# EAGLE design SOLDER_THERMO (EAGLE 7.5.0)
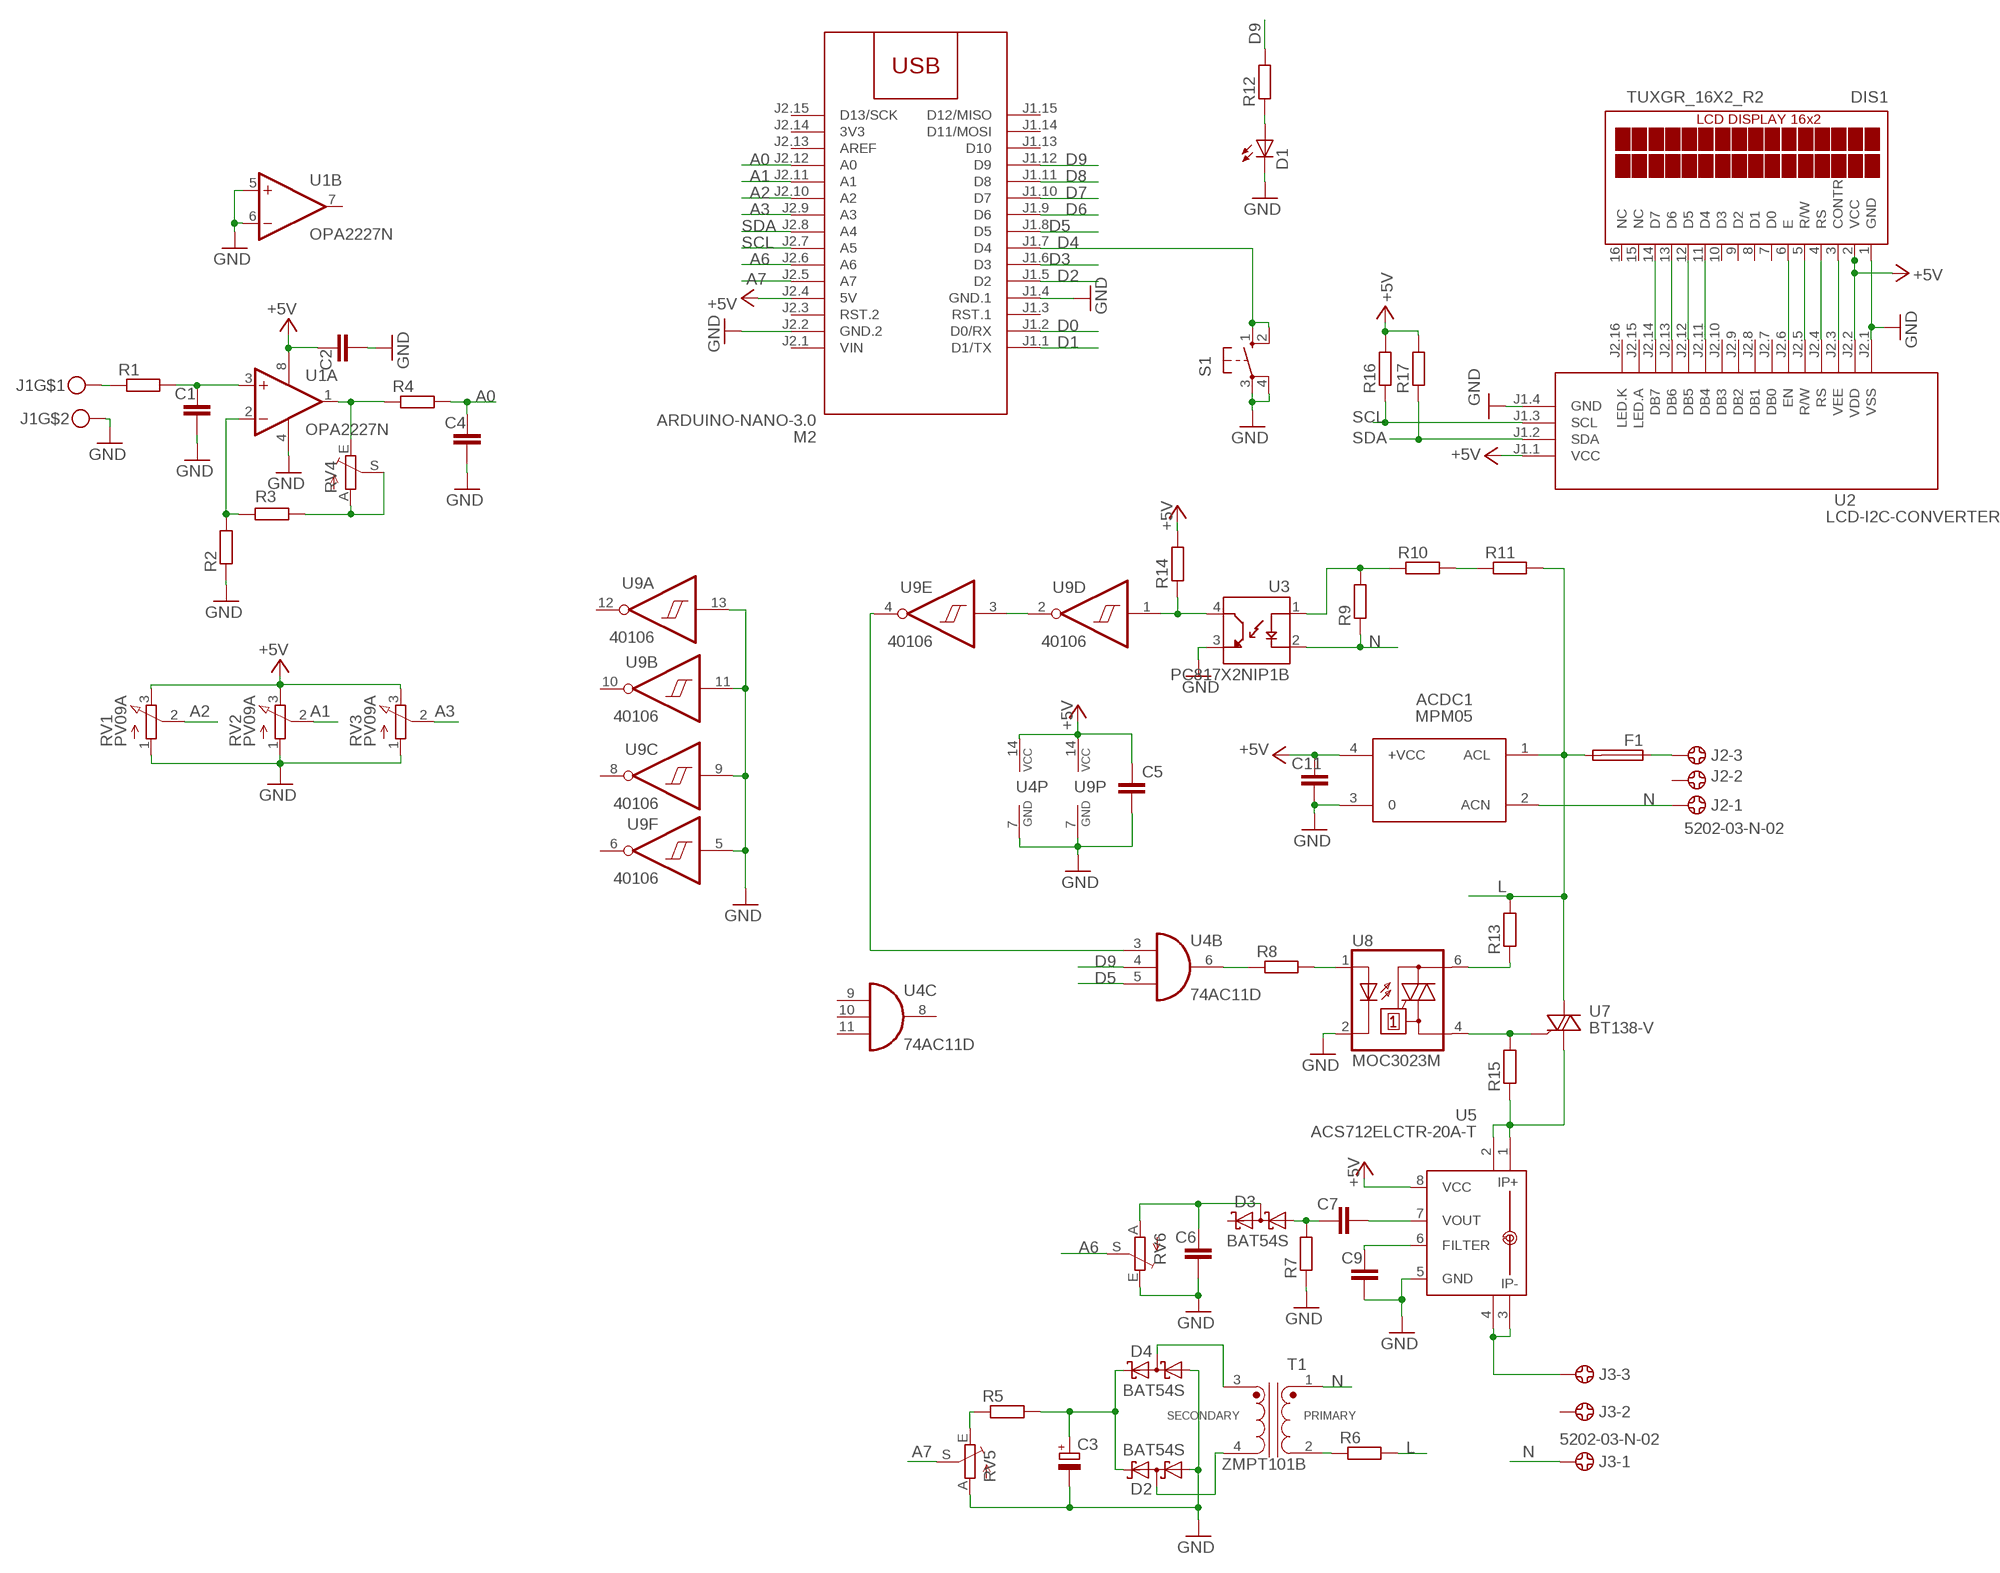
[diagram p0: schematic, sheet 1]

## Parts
ACDC1  MPM05  [MPM05]
C1  C-EUC1206  [C1206]
C2  C-EUC1206  [C1206]
C3  CPOL-EUSMCB  [SMC_B]
C4  C-EUC1206  [C1206]
C5  C-EUC1206  [C1206]
C6  C-EUC1206  [C1206]
C7  C-EUC1206  [C1206]
C9  C-EUC1206  [C1206]
C11  C-EUC1206  [C1206]
D1  LED5MM  [LED5MM]
D2  BAT54S  [SOT23]
D3  BAT54S  [SOT23]
D4  BAT54S  [SOT23]
DIS1  TUXGR_16X2_R2  [TUXGR_16X2_R2]
F1  FUSEBLANK_5X20MM  [FUSE_HOLDER_5X20MM]
J1  MKDSN1,5-2-5,08  [MKDSN1,5-2-5,08]
J2  5202-03-N-02  [5202-03-N-02]
J3  5202-03-N-02  [5202-03-N-02]
M2  ARDUINO-NANO-3.0  [ARDUINO-NANO-3.0]
R1  R-EU_R1206  [R1206]
R2  R-EU_R1206  [R1206]
R3  R-EU_R1206  [R1206]
R4  R-EU_R1206  [R1206]
R5  R-EU_R1206  [R1206]
R6  R-EU_0617/22  [0617/22]
R7  R-EU_R1206  [R1206]
R8  R-EU_R1206  [R1206]
R9  R-EU_R2512  [R2512]
R10  R-EU_R2512  [R2512]
R11  R-EU_R2512  [R2512]
R12  R-EU_R1206  [R1206]
R13  R-EU_R1206  [R1206]
R14  R-EU_R1206  [R1206]
R15  R-EU_R1206  [R1206]
R16  R-EU_R1206  [R1206]
R17  R-EU_R1206  [R1206]
RV1  PV09A  [PTV09]
RV2  PV09A  [PTV09]
RV3  PV09A  [PTV09]
RV4  TRIM_EU-B64W  [B64W]
RV5  TRIM_EU-B64W  [B64W]
RV6  TRIM_EU-B64W  [B64W]
S1  10-XX  [B3F-10XX]
T1  ZMPT101B  [XFMR_ZMPT101B]
U1  OPA2227N  [DIL08]
U2  LCD-I2C-CONVERTER  [LCD-I2C-CONVERTER]
U3  PC817X2NIP1B  [SOIC254P960X420-4N]
U4  74AC11D  [SO14]
U5  ACS712ELCTR-20A-T  [SO8]
U7  BT138-V  [TO220BV]
U8  MOC3023M  [DIL06]
U9  40106  74HC14D  [SO14]

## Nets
+5V: ACDC1.4(+VCC) C2.1 C5.1 C11.1 DIS1.2(VCC) M2.J2.4(5V) R14.2 R16.2 R17.2 RV1.3(E) RV2.3(E) RV3.3(E) U1.8(P:V+) U2.J1.1(VCC) U2.J2.2(VDD) U4.14(P:VCC) U5.8(VCC) U9.14(P:VCC)
A0: C4.1 M2.J2.12(A0) R4.2
A1: M2.J2.11(A1) RV2.2(S)
A2: M2.J2.10(A2) RV1.2(S)
A3: M2.J2.9(A3) RV3.2(S)
A6: M2.J2.6(A6) RV6.S
A7: M2.J2.5(A7) RV5.S
D0: M2.J1.2(D0/RX)
D1: M2.J1.1(D1/TX)
D2: M2.J1.5(D2)
D3: M2.J1.6(D3)
D4: M2.J1.7(D4) S1.1(S) S1.2(S1)
D5: M2.J1.8(D5) U4.5(B:I2)
D6: M2.J1.9(D6)
D7: M2.J1.10(D7)
D8: M2.J1.11(D8)
D9: M2.J1.12(D9) R12.2 U4.4(B:I1)
GND: ACDC1.3 C1.2 C2.2 C3.- C4.2 C5.2 C6.2 C9.2 C11.2 D1.K(C) D2.1(A1) D4.1(A1) DIS1.1(GND) J1.2 M2.J1.4(GND.1) M2.J2.2(GND.2) R2.1 R7.1 RV1.1(A) RV2.1(A) RV3.1(A) RV5.A RV6.E S1.3(P) S1.4(P1) U1.4(P:V-) U1.5(B:+IN) U1.6(B:-IN) U2.J1.4(GND) U2.J2.1(VSS) U3.3(ET) U4.7(P:GND) U5.5(GND) U8.2(C) U9.5(F:I) U9.7(P:GND) U9.9(C:I) U9.11(B:I) U9.13(A:I)
L: ACDC1.1(ACL) F1.2 R6.2 R11.2 R13.2 U7.T2(A2)
N: ACDC1.2(ACN) J2.1 J3.1 R9.1 T1.1 U3.2(C)
N$1: DIS1.14(D7) U2.J2.14(DB7)
N$2: DIS1.13(D6) U2.J2.13(DB6)
N$3: DIS1.12(D5) U2.J2.12(DB5)
N$4: DIS1.11(D4) U2.J2.11(DB4)
N$5: DIS1.6(E) U2.J2.6(EN)
N$6: DIS1.5(R/W) U2.J2.5(R/W)
N$7: DIS1.4(RS) U2.J2.4(RS)
N$8: R2.2 R3.2 U1.2(A:-IN)
N$9: C1.1 R1.2 U1.3(A:+IN)
N$10: DIS1.3(CONTR) U2.J2.3(VEE)
N$11: U9.2(D:O) U9.3(E:I)
N$12: R3.1 RV4.A RV4.S
N$13: R4.1 RV4.E U1.1(A:OUT)
N$14: J1.1 R1.1
N$15: R9.2 R10.1 U3.1(A)
N$16: R10.2 R11.1
N$17: R14.1 U3.4(CT) U9.1(D:I)
N$18: R8.2 U8.1(A)
N$19: F1.1 J2.3
N$20: R6.1 T1.2
N$21: R13.1 U8.6(A2)
N$23: R15.2 U7.G U8.4(A1)
N$24: R15.1 U5.1(IP+) U5.2(IP+1) U7.T1(A1)
N$25: R8.1 U4.6(B:O)
N$26: U4.3(B:I0) U9.4(E:O)
N$27: C9.1 U5.6(FILTER)
N$28: D4.3(C1A2) T1.3
N$29: D2.3(C1A2) T1.4
N$30: C3.+ D2.2(C2) D4.2(C2) R5.2
N$31: J3.3 U5.3(IP-) U5.4(IP-1)
N$32: C7.2 U5.7(VOUT)
N$33: C7.1 D3.1(A1) R7.2
N$34: C6.1 D3.3(C1A2) RV6.A
N$35: R5.1 RV5.E
N$37: D1.A R12.1
SCL: M2.J2.7(A5) R16.1 U2.J1.3(SCL)
SDA: M2.J2.8(A4) R17.1 U2.J1.2(SDA)
Unconnected: D3.2(C2) DIS1.7(D0) DIS1.8(D1) DIS1.9(D2) DIS1.10(D3) DIS1.15(NC) DIS1.16(NC) J2.2 J3.2 M2.J1.3(RST.1) M2.J1.13(D10) M2.J1.14(D11/MOSI) M2.J1.15(D12/MISO) M2.J2.3(RST.2) M2.J2.13(AREF) M2.J2.15(D13/SCK) U1.7(B:OUT) U2.J2.7(DB0) U2.J2.8(DB1) U2.J2.9(DB2) U2.J2.10(DB3) U2.J2.15(LED.A) U2.J2.16(LED.K) U4.1(A:I0) U4.2(A:I1) U4.8(C:O) U4.9(C:I0) U4.10(C:I1) U4.11(C:I2) U4.12(A:O) U4.13(A:I2) U9.6(F:O) U9.8(C:O) U9.10(B:O) U9.12(A:O)

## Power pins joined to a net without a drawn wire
3V3: M2.J2.14(3V3)
VIN: M2.J2.1(VIN)

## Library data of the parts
ACDC1 = acdc:MPM05: AC DC Converter 5W
C1 C2 C4-C7 C9 C11 = rcl:C-EU: CAPACITOR, European symbol
C3 = rcl:CPOL-EU: POLARIZED CAPACITOR, European symbol
D1 = led:LED: LED
D2-D4 = diode:BAT54S: Schottky Diodes Pin connection corrected 2011-05-04 Source: Fairchild .. BAT54.pdf
DIS1 = display-lcd:TUXGR_16X2_R2: Tuxgraphics LCD display 16x2 characters reflective, without background light Source: tuxgr_12x2_r2.pdf; OC_FARNELL: unknown; OC_NEWARK: unknown
F1 = fuse:FUSE: Fuse; OC_FARNELL: unknown; OC_NEWARK: unknown
J1 = con-phoenix-508:MKDSN1,5-2-5,08
J2 J3 = con-ebyelectro:5202-03-N-02: Barrier Blocks Sreies 5202 Source: http://www.ebyelectro.com/PDF/5202-XX-N-02.pdf; OC_FARNELL: unknown; OC_NEWARK: unknown
M2 = diy-modules:ARDUINO-NANO-3.0: Arduino Nano 3.0 and compatible devices More details available here: https://www.arduino.cc/en/Main/ArduinoBoardNano Click here to find device on ebay.com
R1-R17 = rcl:R-EU_: RESISTOR, European symbol
RV1-RV3 = pot:PV09A
RV4-RV6 = pot:TRIM_EU-: POTENTIOMETER
S1 = switch-omron:10-XX: OMRON SWITCH; MPN: B3F-1000; OC_FARNELL: 176432; OC_NEWARK: 36M3542
T1 = ZMPT101B:ZMPT101B: Check availability; AVAILABILITY: Not in stock; CHECK_PRICES: https://www.snapeda.com/parts/ZMPT101B/Qingxian+Zeming+Langxi+Electronic/view-part/?ref=eda; DESCRIPTION: Current-type Voltage Transformer; MF: Qingxian Zeming Langxi Electronic; MP: ZMPT101B; PACKAGE: None; PRICE: None; SNAPEDA_LINK: https://www.snapeda.com/parts/ZMPT101B/Qingxian+Zeming+Langxi+Electronic/view-part/?ref=snap
U1 = linear:OPA222*: High Precision, Low Noise OPERATIONAL AMPLIFIERS Source: http://focus.ti.com/lit/ds/symlink/opa227.pdf
U2 = diy-modules:LCD-I2C-CONVERTER: I2C Bus to 4-Bit Parallel LCD Interface with LED backlight driver
U3 = PC817X2NIP1B:PC817X2NIP1B: Check availability; AVAILABILITY: In Stock; CHECK_PRICES: https://www.snapeda.com/parts/PC817X2NIP1B/Sharp/view-part/?ref=eda; DESCRIPTION: Optocoupler DC-IN 1-CH Transistor DC-OUT 4-Pin DIP SMD T/R; MF: Sharp Microelectronics; MP: PC817X2NIP1B; PACKAGE: SMD-4 Sharp Microelectronics; PRICE: None; SNAPEDA_LINK: https://www.snapeda.com/parts/PC817X2NIP1B/Sharp/view-part/?ref=snap
U4 = 74xx-eu:74*11: Triple 3-input AND gate
U5 = allegro:ACS712ELCTR-20A-T: Fully Integrated, Hall Effect-Based Linear Current Sensor with High Voltage Isolation and a Low-Resistance Current Conductor.
U7 = triac:BT138: TRIAC Source: http://www.semiconductors.philips.com BT138_SERIES_2.pdf
U8 = optocoupler:MOC30*M: RANDOM-PHASE OPTOISOLATORS TRIAC DRIVER OUTPUT Source: http://www.fairchildsemi.com MOC3020-M.pdf; MF: FAIRCHILD SEMICONDUCTOR; MPN: MOC3023-M; OC_FARNELL: 1021367; OC_NEWARK: 72K8896
U9 = 74xx-eu:74*14: Hex schmitt trigger INVERTER

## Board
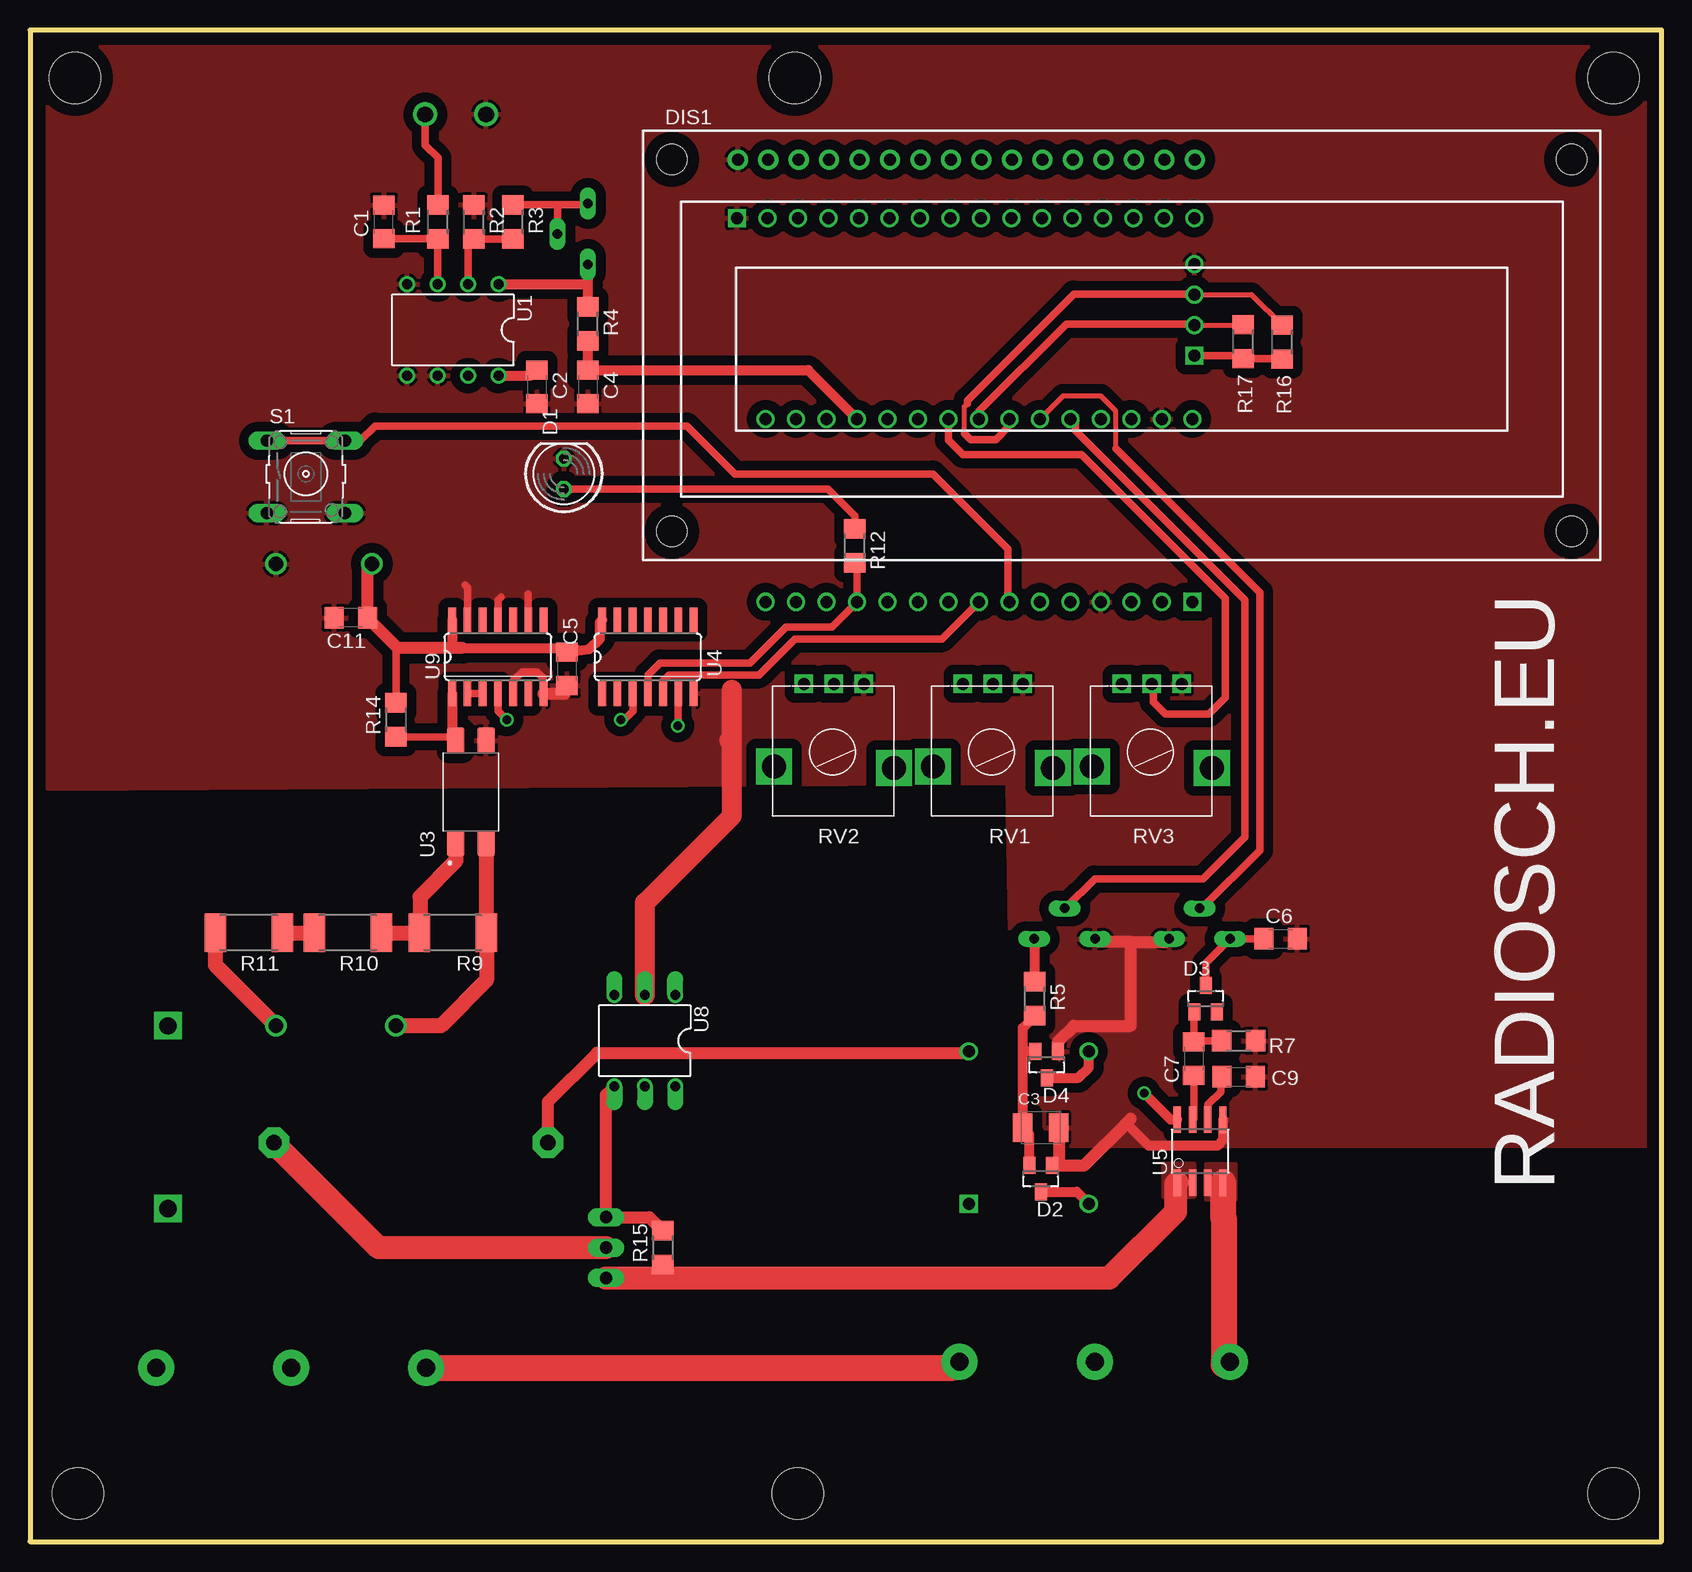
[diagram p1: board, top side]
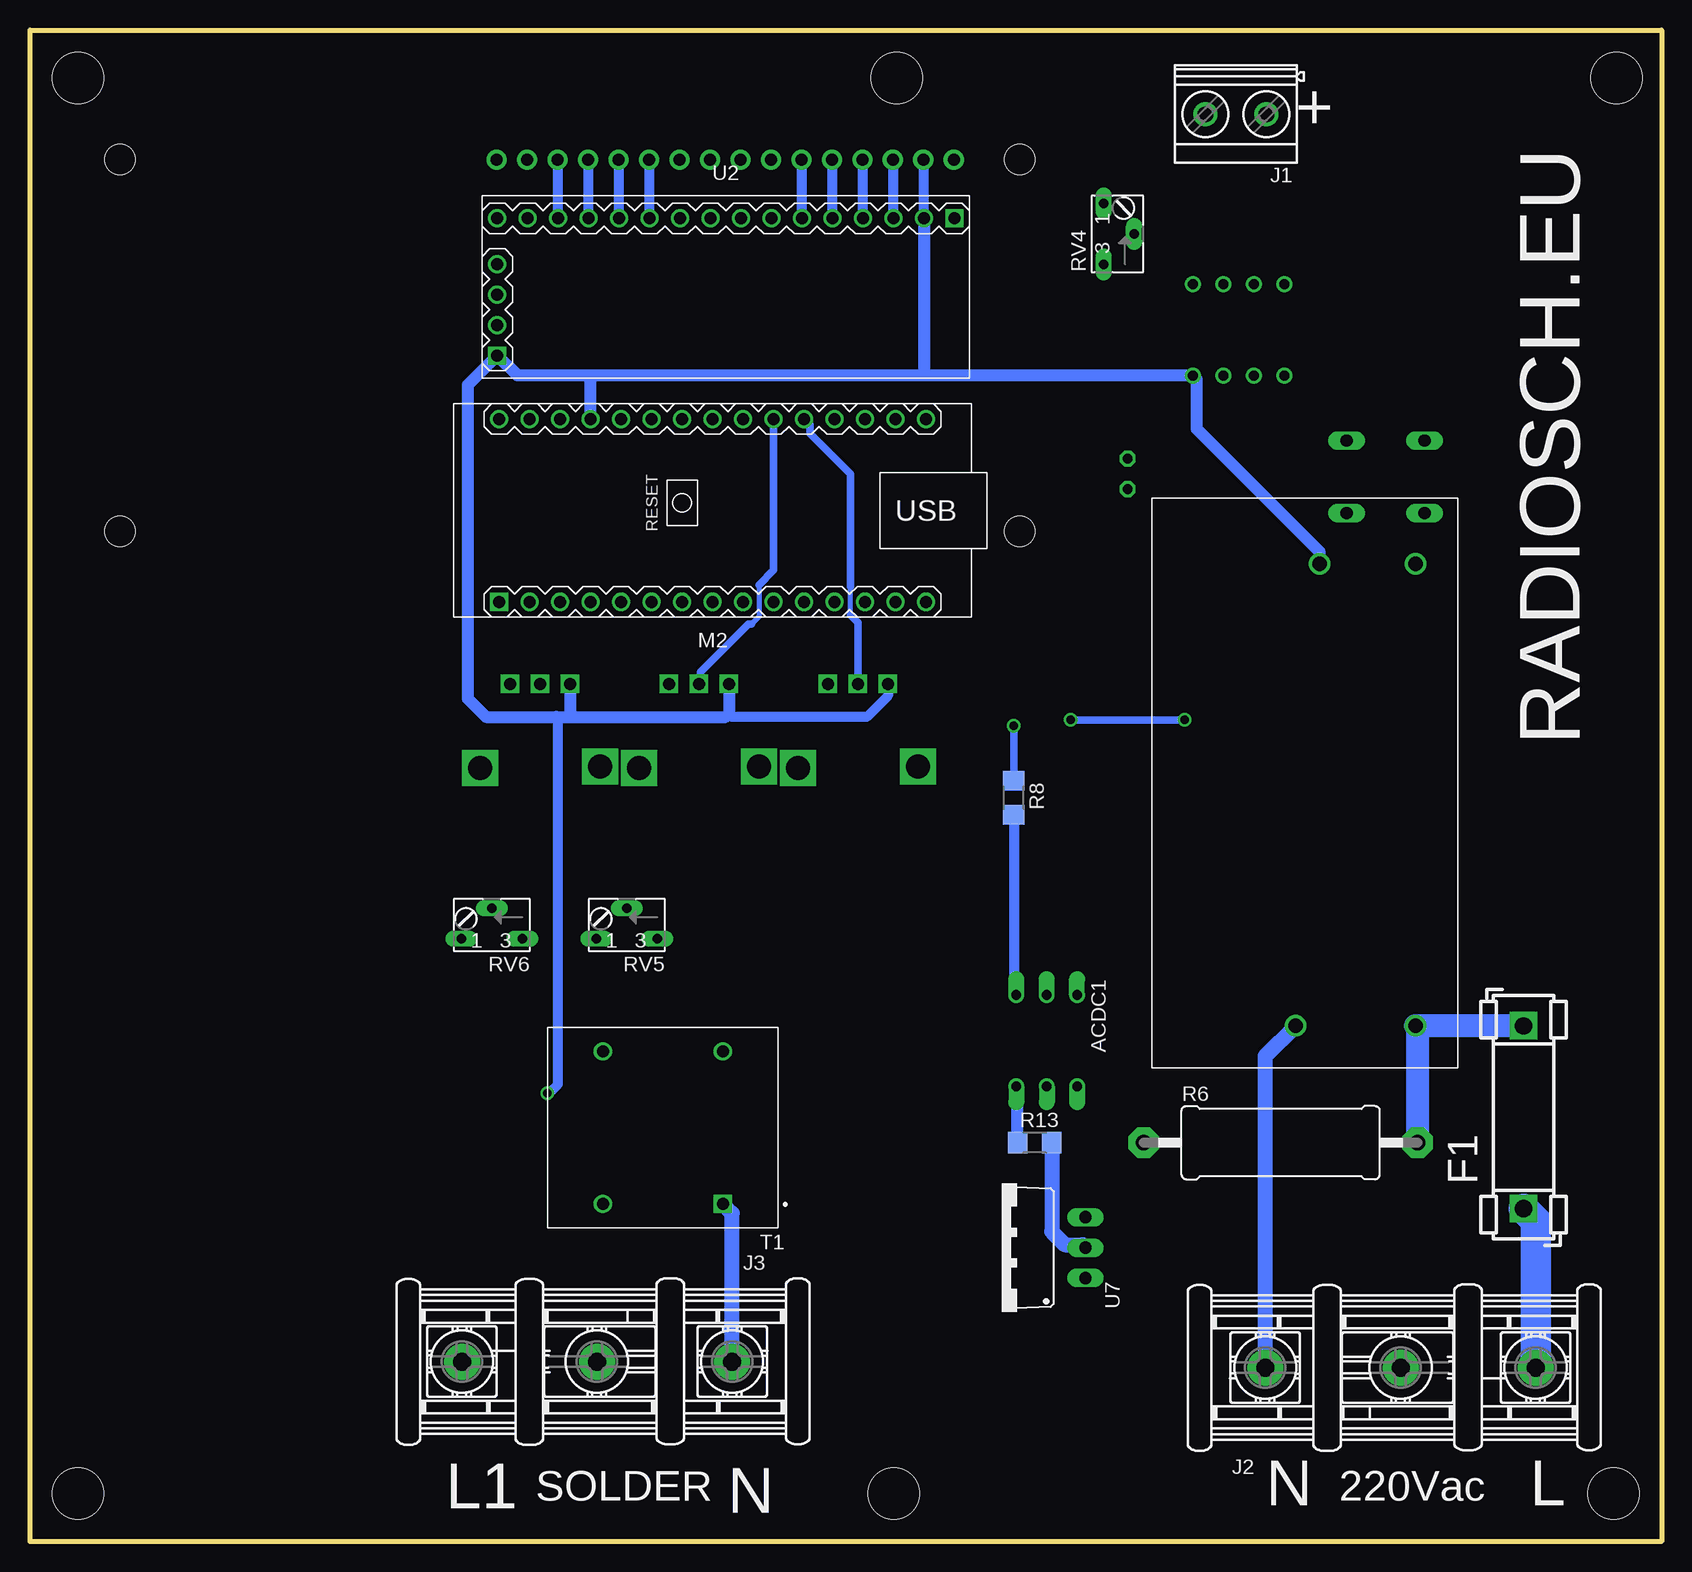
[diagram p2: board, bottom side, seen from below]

Size 136 x 126 mm. Coordinates in mm from the lower left corner, seen from the top.
Outline: 0,0 136,0 136,126 0,126 0,0
Copper layers (1*16): Top 0.035mm / dielectric 1.5mm / Bottom 0.035mm
Design rules "default *": minimum track width 10mil, minimum drill 24mil, track to track 4mil, track to pad 6mil, pad to pad 4mil, via to via 8mil, smd to smd 8mil, copper to edge 40mil, drill to drill 8mil, minimum pad ring 10mil, minimum via ring 8mil, stop-mask expansion 4mil, vias tented up to drill 0mil, thermal gap 10mil
Holes 4.3 mm at 3.75,122 4,4 132,4 132,122 64,4 63.75,122

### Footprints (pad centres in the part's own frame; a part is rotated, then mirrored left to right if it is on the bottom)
MPM05 = drill 1.2: 1 3.5,-22; 2 3.5,-12; 3 42,-22; 4 42,-14
C1206 = smd 1.6 x 1.8: 1 -1.4,0; 2 1.4,0
SMC_B = smd 1.6 x 2.4: + -1.5,0; - 1.5,0
LED5MM = drill 0.813 octagon: A -1.27,0; K 1.27,0
SOT23 = smd 1 x 1.4: 1 -0.95,-1.1; 2 0.95,-1.1; 3 0,1.1
TUXGR_16X2_R2 = drill 1 pad 1.676: 1 -32,15.5; 2 -29.46,15.5; 3 -26.92,15.5; 4 -24.38,15.5; 5 -21.84,15.5; 6 -19.3,15.5; 7 -16.76,15.5; 8 -14.22,15.5; 9 -11.68,15.5; 10 -9.14,15.5; 11 -6.6,15.5; 12 -4.06,15.5; 13 -1.52,15.5; 14 1.02,15.5; 15 3.56,15.5; 16 6.1,15.5 | hole 2.5: -37.5,-15.5; 37.5,-15.5; -37.5,15.5; 37.5,15.5
FUSE_HOLDER_5X20MM = drill 1.422 pad 2.286 square: 1 0,0; 2 15.24,0
MKDSN1,5-2-5,08 = drill 1.3 pad 2: 1 -2.561,0.025; 2 2.519,0.025
5202-03-N-02 = drill 1.5 pad 3: 1 -9.29,0; 2 2,0; 3 13.25,0
ARDUINO-NANO-3.0 = drill 1 square: J1.1 17.78,7.62 | drill 1: J1.2 15.24,7.62; J1.3 12.7,7.62; J1.4 10.16,7.62; J1.5 7.62,7.62; J1.6 5.08,7.62; J1.7 2.54,7.62; J1.8 0,7.62; J1.9 -2.54,7.62; J1.10 -5.08,7.62; J1.11 -7.62,7.62; J1.12 -10.16,7.62; J1.13 -12.7,7.62; J1.14 -15.24,7.62; J1.15 -17.78,7.62; J2.1 17.78,-7.62; J2.2 15.24,-7.62; J2.3 12.7,-7.62; J2.4 10.16,-7.62; J2.5 7.62,-7.62; J2.6 5.08,-7.62; J2.7 2.54,-7.62; J2.8 0,-7.62; J2.9 -2.54,-7.62; J2.10 -5.08,-7.62; J2.11 -7.62,-7.62; J2.12 -10.16,-7.62; J2.13 -12.7,-7.62; J2.14 -15.24,-7.62; J2.15 -17.78,-7.62
R1206 = smd 1.6 x 1.803: 1 -1.422,0; 2 1.422,0
0617/22 = drill 1.3 pad 2.54 octagon: 1 -11.43,0; 2 11.43,0
R2512 = smd 1.8 x 3.2: 1 -2.8,0; 2 2.8,0
PTV09 = drill 1 square: 1 -2.5,0; 2 0,0; 3 2.5,0 | drill 2 square: P$4 -5,7; P$5 5,6.9
B64W = drill 0.813 long: A 2.54,0; E -2.54,0; S 0,-2.54
B3F-10XX = drill 1.016 long: 1 -3.251,2.761; 2 3.251,2.761; 3 -3.251,-3.261; 4 3.251,-3.261
XFMR_ZMPT101B = drill 1 square: 1 -5,6.35 | drill 1: 2 -5,-6.35; 3 5,-6.35; 4 5,6.35
DIL08 = drill 0.813 pad 1.27: 1 -3.81,-3.81; 2 -1.27,-3.81; 3 1.27,-3.81; 4 3.81,-3.81; 5 3.81,3.81; 6 1.27,3.81; 7 -1.27,3.81; 8 -3.81,3.81
LCD-I2C-CONVERTER = drill 1 square: J1.1 -19.05,-5.08; J2.1 19.05,6.35 | drill 1: J1.2 -19.05,-2.54; J1.3 -19.05,0; J1.4 -19.05,2.54; J2.2 16.51,6.35; J2.3 13.97,6.35; J2.4 11.43,6.35; J2.5 8.89,6.35; J2.6 6.35,6.35; J2.7 3.81,6.35; J2.8 1.27,6.35; J2.9 -1.27,6.35; J2.10 -3.81,6.35; J2.11 -6.35,6.35; J2.12 -8.89,6.35; J2.13 -11.43,6.35; J2.14 -13.97,6.35; J2.15 -16.51,6.35; J2.16 -19.05,6.35
SOIC254P960X420-4N = smd 2.15 x 1.48: 1 -4.28,1.27; 2 -4.28,-1.27; 3 4.28,-1.27; 4 4.28,1.27
SO14 = smd 0.66 x 2.032: 1 -3.81,-3.073; 2 -2.54,-3.073; 3 -1.27,-3.073; 4 0,-3.073; 5 1.27,-3.073; 6 2.54,-3.073; 7 3.81,-3.073; 8 3.81,3.073; 9 2.54,3.073; 10 1.27,3.073; 11 0,3.073; 12 -1.27,3.073; 13 -2.54,3.073; 14 -3.81,3.073
SO8 = smd 0.61 x 2.21: 1 0.635,-0.076; 2 1.905,-0.076; 3 3.175,-0.076; 4 4.445,-0.076; 5 4.445,5.156; 6 3.175,5.156; 7 1.905,5.156; 8 0.635,5.156
TO220BV = drill 1.016 long: G 2.54,-6.985; T1 -2.54,-6.985; T2 0,-6.985
DIL06 = drill 0.813 offset: 1 -2.54,-3.81; 2 0,-3.81; 3 2.54,-3.81; 4 2.54,3.81; 5 0,3.81; 6 -2.54,3.81

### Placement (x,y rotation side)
ACDC1  42.5,39.5 90 bottom
C1  29.5,110 90 top
C2  42.25,96.25 270 top
C3  84.25,34.5 0 top
C4  46.5,96.25 270 top
C5  44.75,72.75 270 top
C6  104.25,50.25 0 top
C7  97,40.25 270 top
C9  100.75,38.75 0 top
C11  26.75,77 180 top
D1  44.5,89 90 top
D2  84.25,30.25 180 top
D3  98,45.25 0 top
D4  84.75,39.75 180 top
DIS1  91,99.7 0 top
F1  11.5,27.75 90 bottom
J1  35.5,119 180 bottom
J2  23.75,14.5 0 bottom
J3  86.75,15 180 bottom
M2  79.1,85.95 180 bottom
R1  34,110 270 top
R2  37,110 270 top
R3  40.25,110 270 top
R4  46.5,101.5 270 top
R5  83.75,45.25 270 top
R6  31.75,33.25 0 bottom
R7  100.75,41.75 180 top
R8  54,62 270 bottom
R9  35.25,50.75 180 top
R10  26.5,50.75 180 top
R11  18.25,50.75 180 top
R12  68.75,83 270 top
R13  52.25,33.25 0 bottom
R14  30.5,68.5 90 top
R15  52.75,24.5 90 top
R16  104.38,99.97 270 top
R17  101.12,100.03 270 top
RV1  80.25,71.5 180 top
RV2  67,71.5 180 top
RV3  93.5,71.5 180 top
RV4  46.5,109 90 bottom
RV5  86.25,50.25 180 bottom
RV6  97.5,50.25 180 bottom
S1  23,89 0 top
T1  83.25,34.5 180 bottom
U1  35.25,101 180 top
U2  78,103.95 0 bottom
U3  36.75,62.5 90 top
U4  51.5,73.75 0 top
U5  95,30 0 top
U7  55,24.5 90 bottom
U8  51.25,41.75 180 top
U9  39,73.75 0 top

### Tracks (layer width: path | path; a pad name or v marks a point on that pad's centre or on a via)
+5V  (via drill 0.7)
  Top 0.61: U2.J1.1 100.86,98.87 R17.2 104.33,98.6 R16.2 | R14.2 30.5,74.35 30.65,74.5
  Top 0.813: U9.14 35.19,74.69 35,74.5 | 36,74.5 45.4,74.5 C5.1 46.65,74.4 47.5,75.25 47.5,76.63 U4.14 | U1.8 41.79,97.19 C2.1 | U5.8 95.09,35.16 v92.88,37.38
  Top 1.016: ACDC1.4 28.15,81.15 C11.1 30.65,74.5 35,74.5 36,74.5
  Bottom 0.813: U2.J2.2 61.49,115.15 DIS1.2 | RV2.3 64.5,70.5 66.25,68.75 77.5,68.75 77.75,69 | v92.88,37.38 92.75,37.38 92,38.12 92,68.62 92.12,68.75
  Bottom 1.016: 61.25,97.19 U1.8 38.75,96.88 38.75,92.75 28.5,82.5 ACDC1.4 | 61.25,97.19 89,97.19 | 89,97.19 95.37,97.19 U2.J1.1 99.5,96.42 99.5,70.25 98,68.75 92.12,68.75 90.75,68.75 | M2.J2.4 89.26,96.93 89,97.19 | U2.J2.2 61.49,97.43 61.25,97.19 | 90.75,68.75 78,68.75 77.75,69 RV1.3 | RV3.3 91,69 90.75,68.75
A0
  Top 0.813: R4.2 C4.1 64.86,97.65 M2.J2.12
A1
  Bottom 0.406: 67.62,77.25 67.62,79.62
  Bottom 0.61: RV2.2 67,76.62 67.62,77.25 | 67.62,79.62 67.62,89 71,92.38 71,93.09 M2.J2.11
A2
  Bottom 0.406: 75.25,79.75 75.25,77.12 75.88,76.5
  Bottom 0.61: M2.J2.10 74.02,80.98 75.25,79.75 | 75.88,76.5 76.12,76.5 80.12,72.5 80.12,71.62 RV1.2
A3
  Top 0.61: M2.J2.9 76.56,91.81 77.75,90.62 87.62,90.62 99.62,78.62 99.62,70.38 98.25,69 94.62,69 93.62,70 93.62,71.38 RV3.2
A6
  Top 0.406: 90.5,91.12 90.5,94.25 89.25,95.5 86.11,95.5 M2.J2.6
  Top 0.61: 97.66,52.79 102.5,57.62 102.5,79.12 90.5,91.12
  Top 0.813: RV6.S 97.66,52.79
A7
  Top 0.61: RV5.S 86.29,52.79 88.75,55.25 97.75,55.25 101.25,58.75 101.25,78.5 87.12,92.62 87.12,93.17 M2.J2.5
D4
  Top 0.61: M2.J1.7 81.5,78.47 81.5,82.75 75.25,89 58.75,89 54.75,93 28.75,93 27.51,91.76 S1.2 S1.1
D5
  Top 0.61: U4.5 52.77,71.77 53.25,72.25 60.75,72.25 63.75,75.25 76.02,75.25 M2.J1.8
D9
  Top 0.61: U4.4 51.5,72.25 52.5,73.25 60,73.25 63,76.25 66.86,76.25 M2.J1.12 68.94,81.39 R12.2
GND
  Top 0.61: U9.5 40.27,71.77 41,72.5 42.25,72.5 42.75,72 42.75,70.74 U9.7 | U9.13 36.46,79.54 36.25,79.75 | U9.11 39,78.5 39.25,78.75 | U9.9 41.54,78.96 41.5,79
  Top 0.813: U5.5 99.44,33.45 99,33 93.25,33 91.38,34.88
  Top 1.016: D2.1 85.75,31.35 | 85.75,31.35 87.85,31.35 91.38,34.88 91.75,35.25 | 91.75,50 91.75,43 87,43 85.7,41.7 D4.1 | 91.75,50 89.04,50 RV5.A | 91.75,50 94.71,50 RV6.E | C3.- 85.75,31.35 | U9.7 44.58,70.68 C5.2
  Top 1.676: U8.2 51.25,53.25 58.5,60.5 58.5,67 | 58.5,67 58.5,71 | 58.28,66.78 58.5,67
  pour Top (isolate 0.813): 1.5,125.5 135.5,125.5 135.5,33 82,33 81.5,63.25 1.5,62.75
L
  Top 1.27: R11.2 15.45,48.05 ACDC1.1
  Top 1.93: U7.T2 29.07,24.5 R6.2
  Bottom 1.27: R13.2 50.83,25.83 49.75,24.75 48.27,24.75 U7.T2
  Bottom 1.93: R6.2 20.32,42.82 ACDC1.1 F1.2
N
  Top 1.27: U3.2 38.02,50.78 R9.1 38.05,46.8 34.25,43 ACDC1.2
  Top 2.184: J2.1 76.96,14.5 J3.1
  Bottom 1.27: J3.1 77.46,27.36 T1.1 | J2.1 33.04,40.46 ACDC1.2
N$1
  Bottom 0.813: U2.J2.14 91.97,115.15 DIS1.14
N$2
  Bottom 0.813: U2.J2.13 89.43,115.15 DIS1.13
N$3
  Bottom 0.813: U2.J2.12 86.89,115.15 DIS1.12
N$4
  Bottom 0.813: U2.J2.11 84.35,115.15 DIS1.11
N$5
  Bottom 0.813: U2.J2.6 71.65,115.15 DIS1.6
N$6
  Bottom 0.813: U2.J2.5 69.11,115.15 DIS1.5
N$7
  Bottom 0.813: U2.J2.4 66.57,115.15 DIS1.4
N$8
  Top 0.61: U1.2 36.52,108.1 R2.2 R3.2
N$9
  Top 0.61: U1.3 33.98,108.56 R1.2 33.98,108.6 C1.1
N$10
  Bottom 0.813: U2.J2.3 64.03,115.15 DIS1.3
N$11
  Top 0.61: U9.2 U9.3
N$12
  Top 0.61: R3.1 44,111.42 | 44,111.42 46.38,111.42 RV4.A | RV4.S 43.96,111.38 44,111.42
N$13
  Top 0.813: R4.1 46.5,105 | 46.5,105 RV4.E | U1.1 46.31,104.81 46.5,105
N$14
  Top 0.61: R1.1 34,115.35 32.94,116.41 J1.1
N$15
  Top 1.27: U3.1 35.48,56.73 32.5,53.75 32.5,50.8 R9.2 R10.1
N$16
  Top 1.27: R11.1 R10.2
N$17
  Top 0.61: 35.19,67.07 R14.1
  Top 0.813: U9.1 35.19,67.07 U3.4
N$18
  Bottom 0.813: R8.2 54,45.77 U8.1
N$19
  Bottom 2.54: J2.3 10.5,26.75 F1.1
N$20
  Top 1.016: R6.1 43.18,36.68 47.25,40.75 78.15,40.75 T1.2
N$21
  Bottom 1.016: R13.1 53.67,37.82 U8.6
N$23
  Top 1.016: R15.2 51.63,27.04 U7.G 48.02,37.24 U8.4
N$24
  Top 1.016: R15.1 52.75,22.46 52.25,21.96
  Top 1.93: U7.T1 52.25,21.96 89.96,21.96 95.5,27.5 95.5,29.79 U5.1
  pour Top (no thermals): 94.5,31.5 97,31.5 97,28.75 94.5,28.75
N$25  (via drill 0.7)
  Top 0.61: U4.6 54.04,68.04 v54,68
  Bottom 0.61: v54,68 R8.1
N$26  (via drill 0.7)
  Top 0.61: U9.4 39,69.25 v39.75,68.5 | U4.3 50.25,70.66 50.25,69.25 49.5,68.5 v49.25,68.5
  Bottom 0.61: v39.75,68.5 v49.25,68.5
N$27
  Top 0.61: U5.6 98.17,36.42 99.25,37.5 99.25,38.65 C9.1
N$28
  Top 0.813: D4.3 87.4,38.65 88.25,39.5 T1.3
N$29
  Top 0.813: D2.3 87.25,29.15 T1.4
N$30
  Top 0.813: 82.75,40.75 C3.+ 83.3,33.95 D2.2 | 82.75,40.75 82.75,42.83 R5.2 | D4.2 82.85,40.85 82.75,40.75
N$31
  Top 1.016: 99.44,27.05 99.5,27
  Top 2.184: U5.4 99.44,27.05 | 99.5,27 99.5,14.75 99.75,14.75 J3.3
  pour Top (no thermals): 98,31.5 100.5,31.5 100.5,28.5 98,28.5
N$32
  Top 0.61: C7.2 97,35.25 U5.7
N$33
  Top 0.61: D3.1 97,44.1 C7.1 97.1,41.75 R7.2
N$34
  Top 0.61: D3.3 98,48.21 RV6.A C6.1
N$35
  Top 0.813: R5.1 83.75,50.21 RV5.E
N$37
  Top 0.61: D1.A 66.52,87.73 68.75,85.5 R12.1
SCL
  Top 0.406: U2.J1.3 101.82,103.95 R16.1 | 77.88,92.38 77.88,94.62 78.12,94.88
  Top 0.61: M2.J2.7 81.64,93.02 80.5,91.88 78.38,91.88 77.88,92.38 | 78.12,94.88 78.12,95.12 87,104 97,104 U2.J1.3
SDA
  Top 0.406: U2.J1.2 101.09,101.41 R17.1
  Top 0.61: M2.J2.8 79.1,94.22 86.38,101.5 96.96,101.5 U2.J1.2

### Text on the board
tPlace: RADIOSCH.EU
bPlace: + | RADIOSCH.EU | L | 220Vac | N | SOLDER | L1 | N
